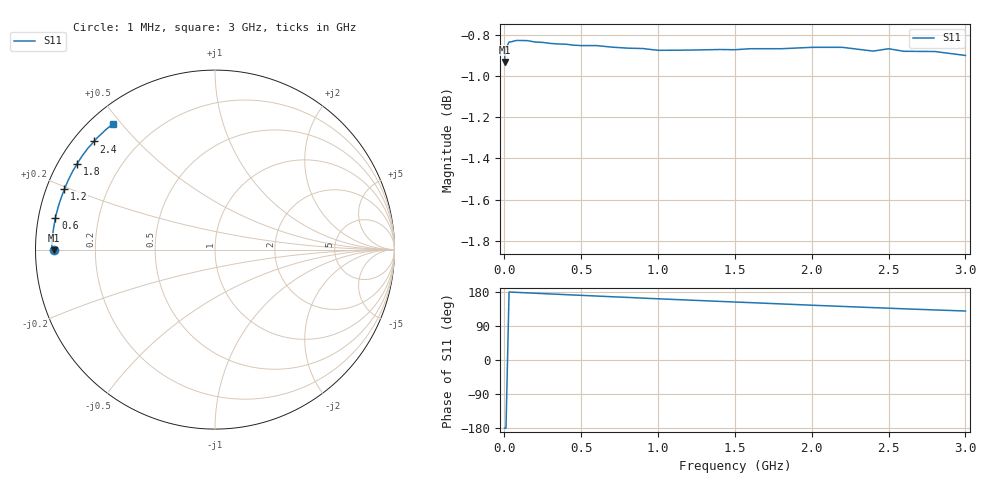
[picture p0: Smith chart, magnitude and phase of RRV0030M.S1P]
! SIEMENS Small Signal Semiconductors
! BA595
! Si PIN Diode in SOD323
! IF = 30 mA
! S-Parameters:  July  1992
# GHz  S  MA  R  50
!  f  S11
! GHz  MAG  ANG
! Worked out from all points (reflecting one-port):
!   33 points, 1 MHz to 3 GHz, reference 50 ohm
!   lowest |S11| = -0.9 dB at 1 MHz (marker M1), VSWR 18.67, Z = 2.68 - j0.131 ohm
!   phase of S11 starts at -180 deg and turns -51 deg over the sweep
!   S11 on the Smith chart (normalised r, x): 1 MHz: 0.05, -0.00; 600 MHz: 0.05, +0.10; 1.2 GHz: 0.05, +0.19; 1.8 GHz: 0.05, +0.29; 2.4 GHz: 0.06, +0.38; 3 GHz: 0.06, +0.47
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0.001  0.8983 -179.7
0.003  0.9026 -179.7
0.01  0.9052 -179.9
0.03  0.9084 179.5
0.08  0.9092 178.5
0.15  0.9091 177.1
0.2  0.9084 176.2
0.25  0.9082 175.2
0.35  0.9074 173.4
0.4  0.9073 172.4
0.5  0.9066 170.6
0.6  0.9066 168.8
0.7  0.9058 166.9
0.8  0.9053 165.2
0.9  0.9051 163.3
1  0.9042 161.5
1.2  0.9043 158.1
1.4  0.9046 154.7
1.5  0.9045 153.0
1.6  0.905 151.4
1.8  0.905 148.0
2  0.9057 144.6
2.2  0.9057 141.4
2.4  0.9038 138.2
2.5  0.905 136.7
2.6  0.9037 135.1
2.8  0.9036 132.1
3  0.9016 129.3
